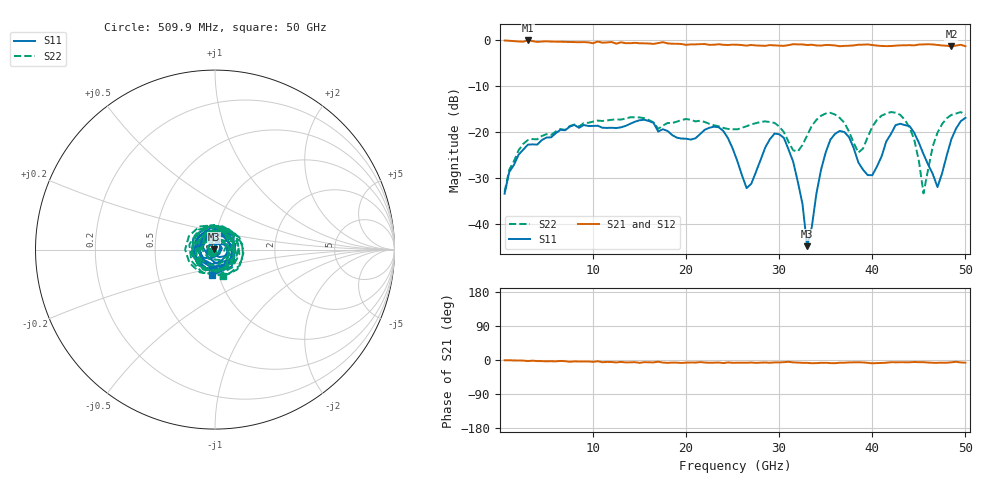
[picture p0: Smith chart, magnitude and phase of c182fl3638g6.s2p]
! 8/5/2019 2:05:06 PM
! Z:\MATT MILLER ENGINEERING\C182FL3638G6.S2P
! CHANNEL.1
! TR.MEASUREMENT
! CORRECTED.DATA
# GHZ S RI R 50.0
! FREQ.GHZ  S11RE  S11IM  S21RE  S21IM  S12RE  S12IM  S22RE  S22IM
!; PortSelection: Port_12
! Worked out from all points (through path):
!   100 points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, 509.9 MHz to 50 GHz, reference 50 ohm
!   highest |S21| = -0.01 dB at 3.009 GHz (marker M1); lowest = -1.3 dB at 48.5 GHz (marker M2)
!   lowest |S11| = -44.7 dB at 33 GHz (marker M3), VSWR 1.01, Z = 49.5 + j0.258 ohm
!   |S11| at or under -10 dB: start of sweep to end of sweep
!   |S22| runs from -33.3 to -15.6 dB; largest |S21 - S12| = 0.038
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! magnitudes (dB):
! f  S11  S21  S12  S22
! 509.9 MHz  -33.3  0.0  0.0  -32.9
! 3.009 GHz  -22.7  0.0  0.0  -21.6
! 9.008 GHz  -18.4  -0.4  -0.3  -18.0
! 17.51 GHz  -19.3  -0.4  -0.5  -18.5
! 23.51 GHz  -18.9  -0.8  -0.8  -18.7
! 25.5 GHz  -26.2  -0.9  -1.0  -19.3
! 26.5 GHz  -32.1  -1.1  -1.1  -18.6
! 29 GHz  -21.5  -1.0  -1.1  -17.7
! 30.5 GHz  -21.2  -1.2  -1.1  -19.9
! 32 GHz  -30.8  -0.9  -0.9  -24.1
! 33 GHz  -44.7  -1.0  -0.9  -20.7
! 33.5 GHz  -40.5  -0.9  -0.9  -18.5
! 34.5 GHz  -28.0  -1.1  -1.1  -16.4
! 36 GHz  -20.3  -1.1  -1.2  -16.1
! 38.5 GHz  -26.5  -0.9  -0.9  -24.4
! 40 GHz  -29.3  -1.0  -1.0  -18.8
! 42 GHz  -20.3  -1.2  -1.1  -15.6
! 44 GHz  -18.6  -1.0  -1.1  -18.9
! 45.5 GHz  -24.7  -0.9  -0.8  -33.3
! 47 GHz  -31.9  -1.0  -0.9  -20.0
! 48.5 GHz  -21.4  -1.3  -1.1  -16.2
! 50 GHz  -16.8  -1.2  -1.4  -16.1
